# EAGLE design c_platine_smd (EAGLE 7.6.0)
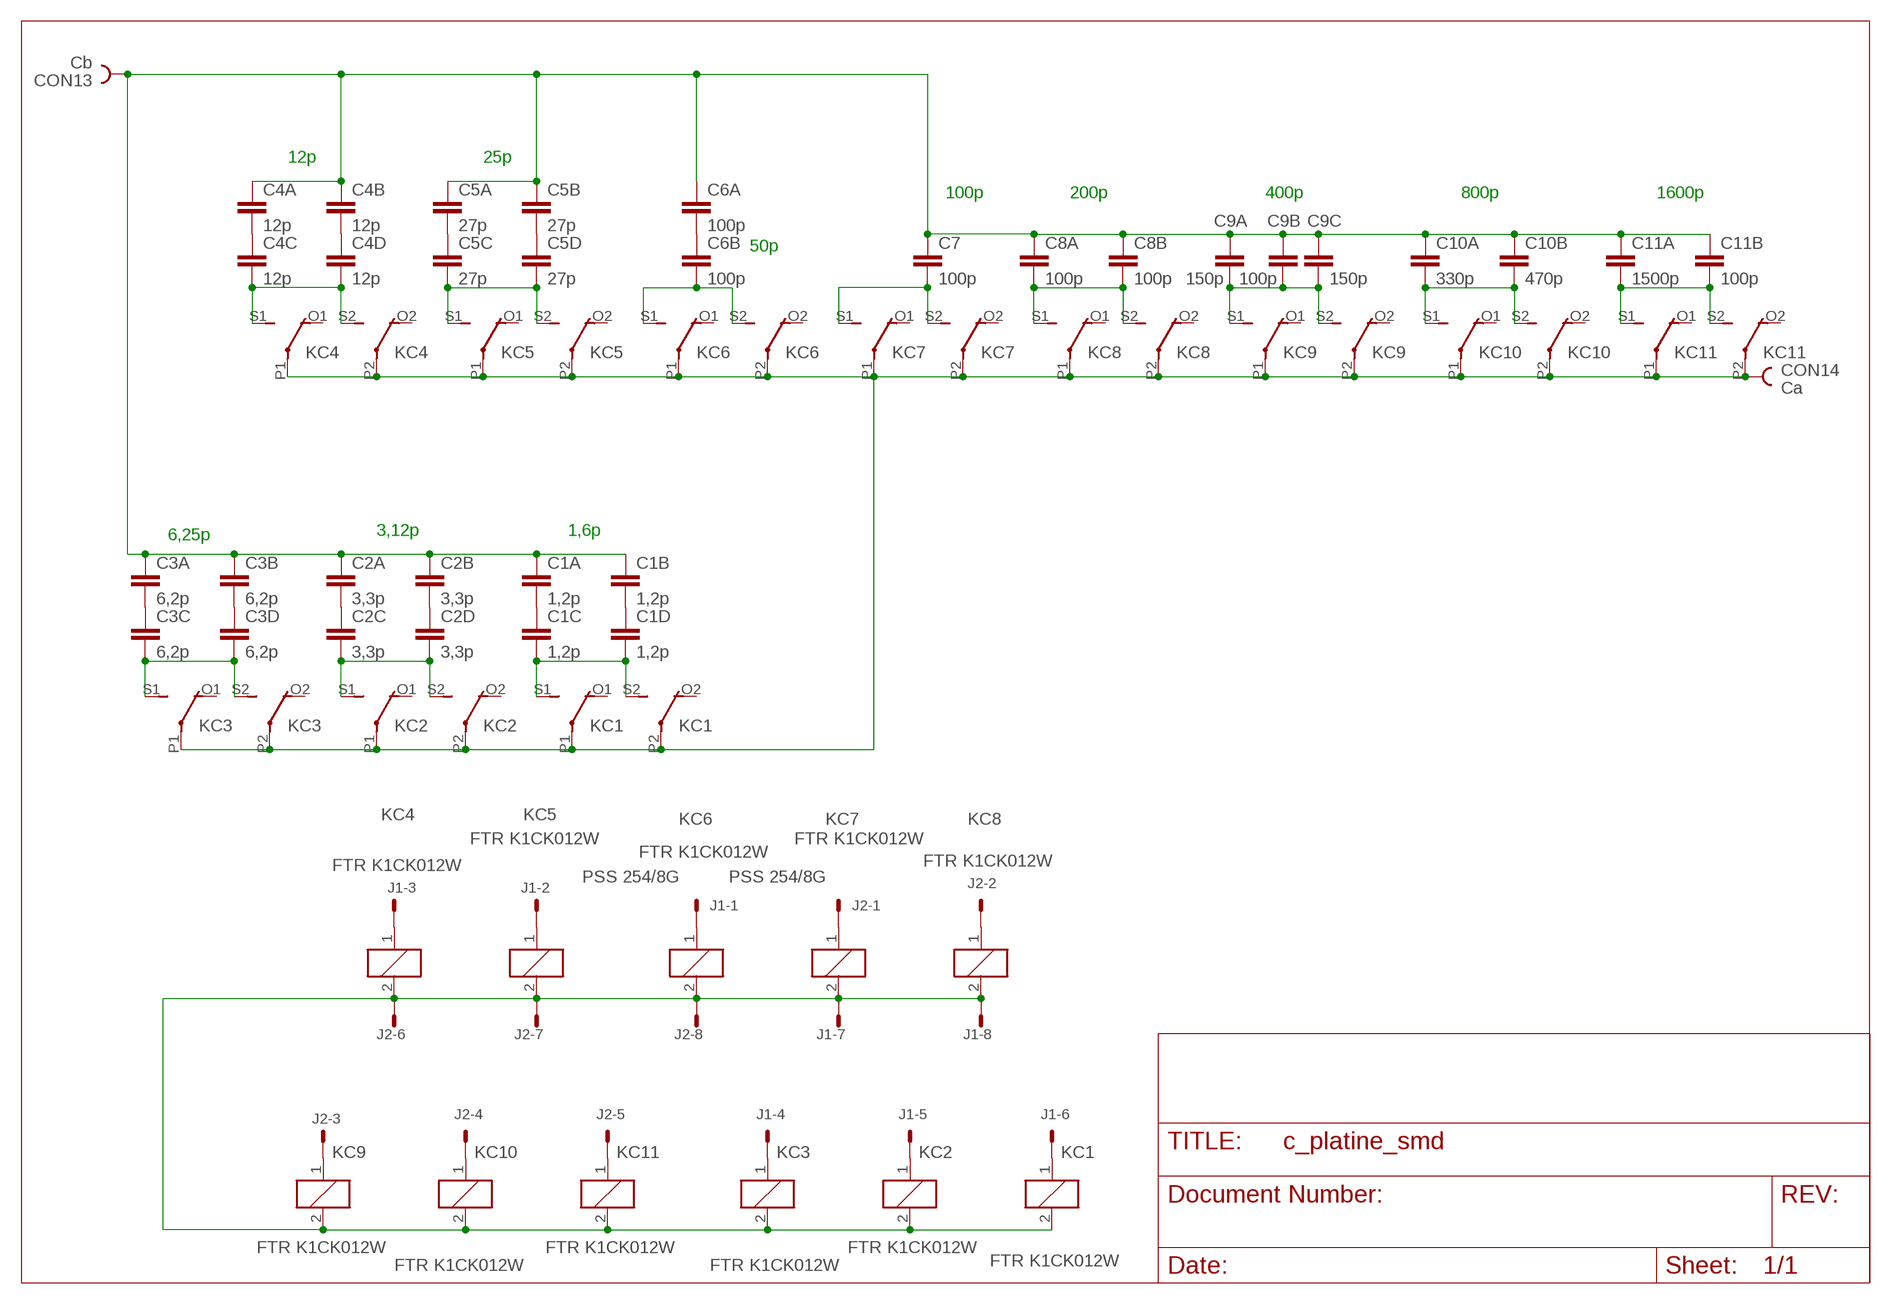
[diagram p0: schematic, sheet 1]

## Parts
C1A  1,2p  C-EUC1812K  [C1812K]
C1B  1,2p  C-EUC1812K  [C1812K]
C1C  1,2p  C-EUC1812K  [C1812K]
C1D  1,2p  C-EUC1812K  [C1812K]
C2A  3,3p  C-EUC1812K  [C1812K]
C2B  3,3p  C-EUC1812K  [C1812K]
C2C  3,3p  C-EUC1812K  [C1812K]
C2D  3,3p  C-EUC1812K  [C1812K]
C3A  6,2p  C-EUC1812K  [C1812K]
C3B  6,2p  C-EUC1812K  [C1812K]
C3C  6,2p  C-EUC1812K  [C1812K]
C3D  6,2p  C-EUC1812K  [C1812K]
C4A  12p  C-EUC1812K  [C1812K]
C4B  12p  C-EUC1812K  [C1812K]
C4C  12p  C-EUC1812K  [C1812K]
C4D  12p  C-EUC1812K  [C1812K]
C5A  27p  C-EUC1812K  [C1812K]
C5B  27p  C-EUC1812K  [C1812K]
C5C  27p  C-EUC1812K  [C1812K]
C5D  27p  C-EUC1812K  [C1812K]
C6A  100p  C-EU150-054X183  [C150-054X183]
C6B  100p  C-EU150-054X183  [C150-054X183]
C7  100p  C-EU150-054X183  [C150-054X183]
C8A  100p  C-EU150-054X183  [C150-054X183]
C8B  100p  C-EU150-054X183  [C150-054X183]
C9A  150p  C-EU150-054X183  [C150-054X183]
C9B  100p  C-EU150-054X183  [C150-054X183]
C9C  150p  C-EU150-054X183  [C150-054X183]
C10A  330p  C-EU150-054X183  [C150-054X183]
C10B  470p  C-EU150-054X183  [C150-054X183]
C11A  1500p  C-EU225-074X268  [C225-074X268]
C11B  100p  C-EU150-054X183  [C150-054X183]
CON13  Cb  PIN2_53MM  [HOLE3]
CON14  Ca  PIN2_53MM  [HOLE3]
J1  PSS 254/8G  22-27-2081-08  [6410-08]
J2  PSS 254/8G  22-27-2081-08  [6410-08]
KC1  FTR K1CK012W  4052  [F4052]
KC2  FTR K1CK012W  4052  [F4052]
KC3  FTR K1CK012W  4052  [F4052]
KC4  FTR K1CK012W  4052  [F4052]
KC5  FTR K1CK012W  4052  [F4052]
KC6  FTR K1CK012W  4052  [F4052]
KC7  FTR K1CK012W  4052  [F4052]
KC8  FTR K1CK012W  4052  [F4052]
KC9  FTR K1CK012W  4052  [F4052]
KC10  FTR K1CK012W  4052  [F4052]
KC11  FTR K1CK012W  4052  [F4052]

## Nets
N$1: CON14.1 KC1.P1(2:P) KC1.P2(3:P) KC2.P1(2:P) KC2.P2(3:P) KC3.P1(2:P) KC3.P2(3:P) KC4.P1(2:P) KC4.P2(3:P) KC5.P1(2:P) KC5.P2(3:P) KC6.P1(2:P) KC6.P2(3:P) KC7.P1(2:P) KC7.P2(3:P) KC8.P1(2:P) KC8.P2(3:P) KC9.P1(2:P) KC9.P2(3:P) KC10.P1(2:P) KC10.P2(3:P) KC11.P1(2:P) KC11.P2(3:P)
N$2: C6A.2 C6B.1
N$3: C5C.2 C5D.2 KC5.S1(2:S) KC5.S2(3:S)
N$4: C6B.2 KC6.S1(2:S) KC6.S2(3:S)
N$5: C7.2 KC7.S1(2:S) KC7.S2(3:S)
N$6: C4C.2 C4D.2 KC4.S1(2:S) KC4.S2(3:S)
N$7: C8A.2 C8B.2 KC8.S1(2:S) KC8.S2(3:S)
N$8: C9A.2 C9B.2 C9C.2 KC9.S1(2:S) KC9.S2(3:S)
N$9: C10A.2 C10B.2 KC10.S1(2:S) KC10.S2(3:S)
N$10: C11A.2 C11B.2 KC11.S1(2:S) KC11.S2(3:S)
N$11: C5A.2 C5C.1
N$12: J1.6 KC1.1
N$13: J1.5 KC2.1
N$14: J1.2 KC5.1
N$15: C4B.2 C4D.1
N$16: J1.7 J1.8 J2.6 J2.7 J2.8 KC1.2 KC2.2 KC3.2 KC4.2 KC5.2 KC6.2 KC7.2 KC8.2 KC9.2 KC10.2 KC11.2
N$17: J1.1 KC6.1
N$18: C5B.2 C5D.1
N$19: J2.1 KC7.1
N$21: J1.4 KC3.1
N$22: J2.5 KC11.1
N$23: J2.3 KC9.1
N$24: J2.4 KC10.1
N$25: J2.2 KC8.1
N$26: J1.3 KC4.1
N$27: C4A.2 C4C.1
N$28: C1A.1 C1B.1 C2A.1 C2B.1 C3A.1 C3B.1 C4A.1 C4B.1 C5A.1 C5B.1 C6A.1 C7.1 C8A.1 C8B.1 C9A.1 C9B.1 C9C.1 C10A.1 C10B.1 C11A.1 C11B.1 CON13.1
N$29: C3C.2 C3D.2 KC3.S1(2:S) KC3.S2(3:S)
N$30: C2C.2 C2D.2 KC2.S1(2:S) KC2.S2(3:S)
N$31: C1C.2 C1D.2 KC1.S1(2:S) KC1.S2(3:S)
N$32: C1B.2 C1D.1
N$33: C2B.2 C2D.1
N$34: C3B.2 C3D.1
N$35: C3A.2 C3C.1
N$36: C2A.2 C2C.1
N$37: C1A.2 C1C.1
Unconnected: KC1.O1(2:O) KC1.O2(3:O) KC2.O1(2:O) KC2.O2(3:O) KC3.O1(2:O) KC3.O2(3:O) KC4.O1(2:O) KC4.O2(3:O) KC5.O1(2:O) KC5.O2(3:O) KC6.O1(2:O) KC6.O2(3:O) KC7.O1(2:O) KC7.O2(3:O) KC8.O1(2:O) KC8.O2(3:O) KC9.O1(2:O) KC9.O2(3:O) KC10.O1(2:O) KC10.O2(3:O) KC11.O1(2:O) KC11.O2(3:O)

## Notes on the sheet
- 12p | 25p
- 100p | 200p | 400p | 800p | 1600p
- 50p
- 6,25p | 3,12p | 1,6p

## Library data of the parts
C1A C1B C1C C1D C2A C2B C2C C2D C3A C3B C3C C3D C4A C4B C4C C4D C5A C5B C5C C5D C6A C6B C7 C8A C8B C9A C9B C9C C10A C10B C11A C11B = rcl:C-EU: CAPACITOR, European symbol
CON13 CON14 = lindenau:PIN2_5
J1 J2 = con-molex:22-?-08: CONNECTOR wire to board 2.54 mm (.1 inch) pitch header; OC_FARNELL: unknown; OC_NEWARK: unknown
KC1-KC11 = relay:4052: RELAY 2 x switch, Finder; OC_FARNELL: unknown; OC_NEWARK: unknown

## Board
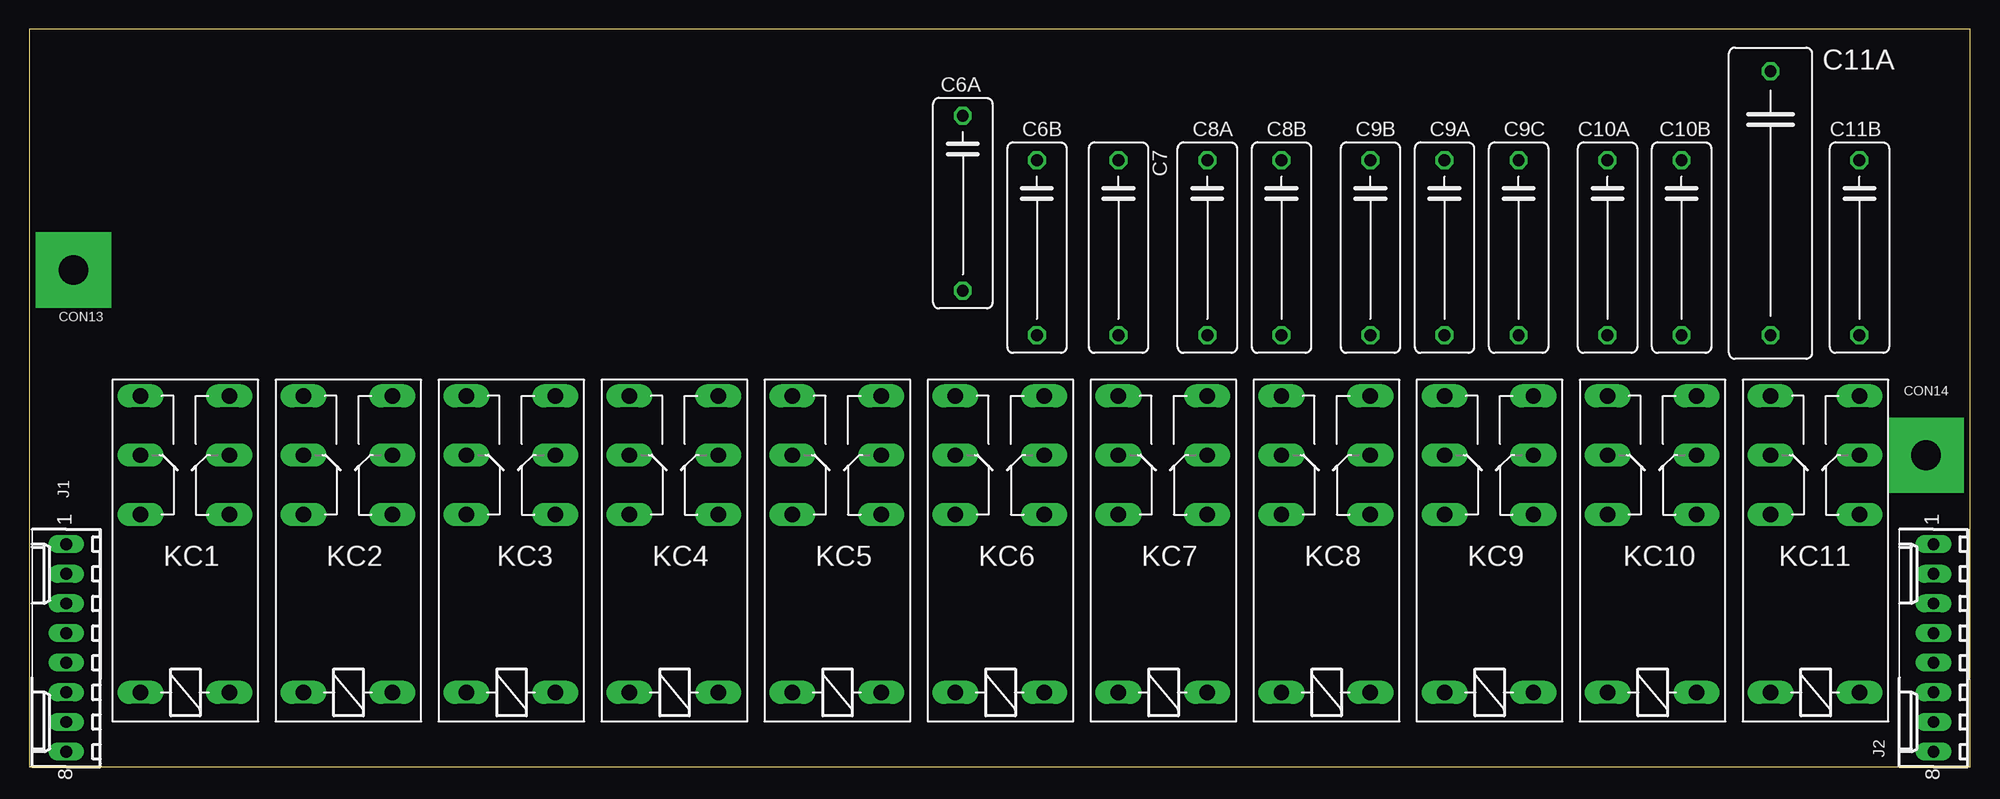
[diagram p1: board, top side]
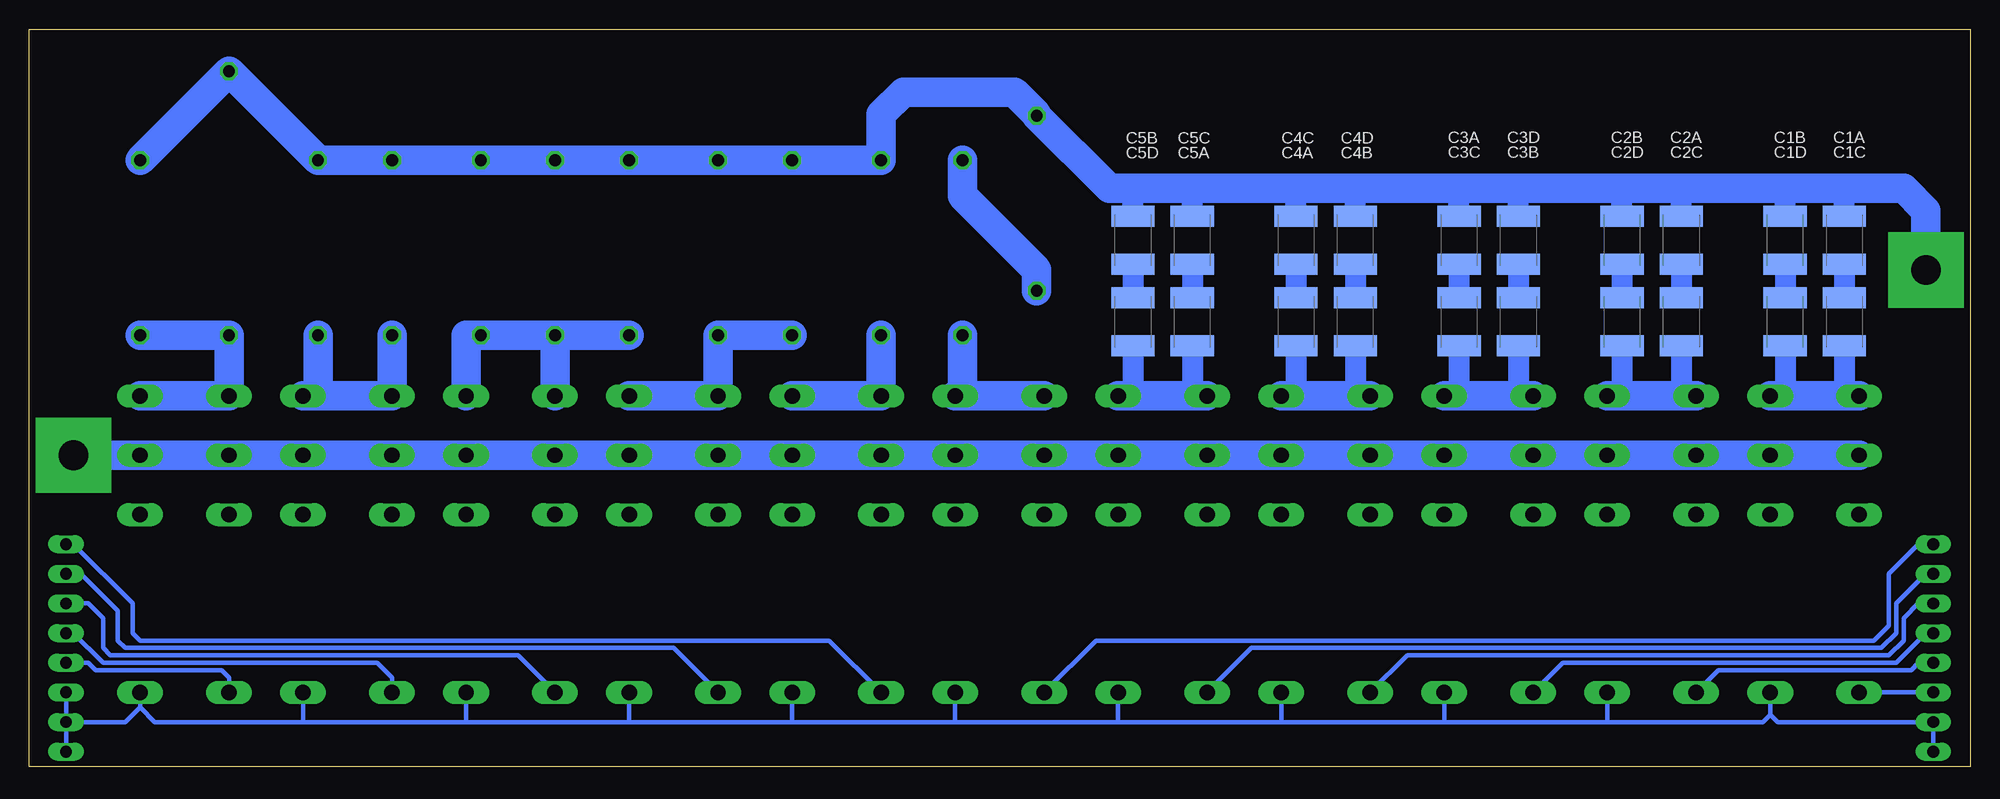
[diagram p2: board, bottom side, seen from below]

Size 166.35 x 63.17 mm. Coordinates in mm from the lower left corner, seen from the top.
Outline: 0,0 166.35,0 166.35,63.17 0,63.17 0,0
Copper layers (1*16): Top 0.035mm / dielectric 1.5mm / Bottom 0.035mm
Design rules "default": minimum track width 10mil, minimum drill 24mil, track to track 8mil, track to pad 8mil, pad to pad 8mil, via to via 8mil, smd to smd 8mil, copper to edge 40mil, drill to drill 8mil, minimum pad ring 10mil, minimum via ring 8mil, stop-mask expansion 4mil, vias tented up to drill 0mil, thermal gap 10mil

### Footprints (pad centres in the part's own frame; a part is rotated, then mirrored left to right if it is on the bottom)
C1812K = smd 1.8 x 3.7: 1 -2.05,0; 2 2.05,0
C150-054X183 = drill 1.016 octagon: 1 -7.493,0; 2 7.493,0
C225-074X268 = drill 1.016 octagon: 1 -11.303,0; 2 11.303,0
HOLE3 = drill 2.54 pad 6.452 square: 1 0,0
6410-08 = drill 1.016 long: 1 8.89,0; 2 6.35,0; 3 3.81,0; 4 1.27,0; 5 -1.27,0; 6 -3.81,0; 7 -6.35,0; 8 -8.89,0
F4052 = drill 1.321 long: 1 -3.81,3.81; 2 -3.81,-3.81; O1 11.43,-3.81; O2 11.43,3.81; P1 16.51,-3.81; P2 16.51,3.81; S1 21.59,-3.81; S2 21.59,3.81

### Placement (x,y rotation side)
C1A  10.79,45.09 270 bottom
C1B  15.88,45.09 270 bottom
C1C  10.79,38.1 270 bottom
C1D  15.88,38.1 270 bottom
C2A  24.77,45.09 270 bottom
C2B  29.85,45.09 270 bottom
C2C  24.77,38.1 270 bottom
C2D  29.85,38.1 270 bottom
C3A  43.81,45.09 270 bottom
C3B  38.73,45.09 270 bottom
C3C  43.81,38.1 270 bottom
C3D  38.73,38.1 270 bottom
C4A  57.78,45.09 270 bottom
C4B  52.7,45.09 270 bottom
C4C  57.78,38.1 270 bottom
C4D  52.7,38.1 270 bottom
C5A  66.67,45.09 270 bottom
C5B  71.75,45.09 270 bottom
C5C  66.67,38.1 270 bottom
C5D  71.75,38.1 270 bottom
C6A  80.01,48.26 270 top
C6B  86.36,44.45 270 top
C7  93.34,44.45 270 top
C8A  100.97,44.45 270 top
C8B  107.31,44.45 270 top
C9A  121.28,44.45 270 top
C9B  114.94,44.45 270 top
C9C  127.63,44.45 270 top
C10A  135.26,44.45 270 top
C10B  141.61,44.45 270 top
C11A  149.23,48.26 270 top
C11B  156.84,44.45 270 top
CON13  3.81,42.55 0 top
CON14  162.56,26.67 0 top
J1  3.17,10.16 90 top
J2  163.2,10.16 90 top
KC1  13.34,10.16 90 top
KC2  27.3,10.16 90 top
KC3  41.27,10.16 90 top
KC4  55.24,10.16 90 top
KC5  69.22,10.16 90 top
KC6  83.19,10.16 90 top
KC7  97.16,10.16 90 top
KC8  111.12,10.16 90 top
KC9  125.09,10.16 90 top
KC10  139.06,10.16 90 top
KC11  153.04,10.16 90 top

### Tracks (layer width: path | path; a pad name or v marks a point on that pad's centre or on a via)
N$1
  Bottom 2.54: KC1.P1 KC1.P2 KC2.P2 KC2.P1 KC3.P2 | KC3.P2 38.73,26.67 | KC3.P2 KC3.P1 KC4.P2 KC4.P1 KC5.P2 KC5.P1 KC6.P2 KC6.P1 KC7.P2 KC7.P1 KC8.P2 KC8.P1 KC9.P2 KC9.P1 KC10.P2 KC10.P1 KC11.P2 KC11.P1 CON14.1
N$2
  Bottom 2.54: C6A.2 80.01,42.55 86.36,48.9 C6B.1
N$3
  Bottom 1.778: C5C.2 66.67,31.75 | C5D.2 71.75,31.75
  Bottom 2.54: KC5.S2 66.67,31.75 70.48,31.75 | 70.48,31.75 71.75,31.75 KC5.S1 | 70.52,31.78 70.48,31.75
N$4
  Bottom 2.54: KC6.S2 84.45,31.75 | 84.45,31.75 86.36,31.75 | 86.36,31.75 KC6.S1 | 84.49,31.78 84.45,31.75 | C6B.2 86.36,31.75
N$5
  Bottom 2.54: C7.2 KC7.S2 KC7.S1
N$6
  Bottom 1.778: C4D.2 52.7,31.75 | C4C.2 57.78,31.75
  Bottom 2.54: KC4.S2 52.7,31.75 56.52,31.75 | 56.52,31.75 57.78,31.75 KC4.S1 | 56.55,31.78 56.52,31.75
N$7
  Bottom 2.54: C8A.2 C8B.2 KC8.S2 KC8.S1
N$8
  Bottom 2.54: C9B.2 C9A.2 | C9A.2 C9C.2 128.91,36.96 KC9.S1 | C9A.2 KC9.S2
N$9
  Bottom 2.54: 141.61,31.75 KC10.S2 C10A.2 | 141.61,31.75 KC10.S1 | 141.61,31.75 C10B.2
N$10
  Bottom 2.54: KC11.S1 KC11.S2 C11A.2 C11B.2
N$11
  Bottom 1.778: C5A.2 C5C.1
N$12
  Bottom 0.406: J1.6 KC1.1
N$13
  Bottom 0.406: J1.5 4.45,8.89 5.08,8.26 21.59,8.26 KC2.1
N$14
  Bottom 0.406: KC5.1 61.59,10.16 7.62,10.16 6.35,11.43 6.35,13.97 3.81,16.51 J1.2
N$15
  Bottom 1.778: C4B.2 C4D.1
N$16
  Bottom 0.406: KC1.2 17.14,4.45 | 17.14,4.45 17.78,3.81 31.12,3.81 | 31.12,3.81 45.08,3.81 | 45.08,3.81 59.05,3.81 | 59.05,3.81 73.02,3.81 | 73.02,3.81 86.99,3.81 | 86.99,3.81 100.97,3.81 | 100.97,3.81 114.94,3.81 | 114.94,3.81 128.91,3.81 | 128.91,3.81 142.88,3.81 | 142.88,3.81 155.58,3.81 156.84,5.08 | 156.84,5.08 KC11.2 | KC10.2 142.88,3.81 | KC9.2 128.91,3.81 | KC8.2 114.94,3.81 | KC7.2 100.97,3.81 | KC6.2 86.99,3.81 | KC5.2 73.02,3.81 | KC4.2 59.05,3.81 | KC3.2 45.08,3.81 | KC2.2 31.12,3.81 | J1.8 J1.7 16.51,3.81 17.14,4.45 | J2.8 J2.7 | J2.7 158.12,3.81 156.84,5.08 | J2.7 J2.6
N$17
  Bottom 0.406: KC6.1 74.93,10.79 8.25,10.79 6.98,12.06 6.98,16.51 4.45,19.05 J1.1
N$18
  Bottom 1.778: C5B.2 C5D.1
N$19
  Bottom 0.406: J2.1 162.56,19.05 157.48,13.97 157.48,11.43 156.84,10.79 97.79,10.79 KC7.1
N$21
  Bottom 0.406: J1.4 3.81,11.43 6.35,8.89 34.92,8.89 KC3.1
N$22
  Bottom 0.406: J2.5 161.29,8.89 160.66,8.26 149.86,8.26 149.23,7.62 KC11.1
N$23
  Bottom 0.406: J2.3 161.29,13.97 160.02,12.7 160.02,10.16 159.39,9.53 124.46,9.53 KC9.1
N$24
  Bottom 0.406: J2.4 162.56,11.43 160.02,8.89 136.53,8.89 135.26,7.62 KC10.1
N$25
  Bottom 0.406: J2.2 161.93,16.51 158.75,13.34 158.75,10.79 158.12,10.16 111.12,10.16 KC8.1
N$26
  Bottom 0.406: KC4.1 48.26,9.53 6.98,9.53 5.71,10.79 5.71,12.7 4.45,13.97 J1.3
N$27
  Bottom 1.778: C4A.2 C4C.1
N$28
  Bottom 1.778: C1A.1 10.79,49.53 | C1B.1 15.88,49.53 | C2A.1 24.77,49.53 | C2B.1 29.85,49.53 | C3B.1 38.73,49.53 | C3A.1 43.81,49.53 | C4B.1 52.7,49.53 | C4A.1 57.78,49.53 | C5A.1 66.67,49.53 | C5B.1 71.75,49.53
  Bottom 2.54: C11B.1 C11A.1 C10B.1 C10A.1 C9C.1 C9A.1 C9B.1 C8B.1 C8A.1 C7.1 93.34,55.88 91.44,57.78 81.91,57.78 80.01,55.88 C6A.1 73.79,49.53 71.75,49.53 66.67,49.53 57.78,49.53 52.7,49.53 43.81,49.53 38.73,49.53 29.85,49.53 24.77,49.53 15.88,49.53 10.79,49.53 5.71,49.53 3.81,47.62 CON13.1
N$29
  Bottom 1.778: C3D.2 38.73,31.75 | C3C.2 43.81,31.75
  Bottom 2.54: KC3.S2 38.73,31.75 43.81,31.75 KC3.S1
N$30
  Bottom 1.778: C2C.2 24.77,31.75 | C2D.2 29.85,31.75
  Bottom 2.54: KC2.S2 24.77,31.75 29.85,31.75 KC2.S1
N$31
  Bottom 1.778: C1C.2 10.79,31.75 | C1D.2 15.88,31.75
  Bottom 2.54: KC1.S2 10.79,31.75 15.88,31.75 KC1.S1
N$32
  Bottom 1.778: C1B.2 C1D.1
N$33
  Bottom 1.778: C2B.2 C2D.1
N$34
  Bottom 1.778: C3B.2 C3D.1
N$35
  Bottom 1.778: C3A.2 C3C.1
N$36
  Bottom 1.778: C2A.2 C2C.1
N$37
  Bottom 1.778: C1A.2 C1C.1

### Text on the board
tDocu: 50p | 100p | 200p | 400p | 800p | 1600p | 1,6p | 3,12p | 6,3p | 12,5p | 25p | KC6 | KC7 | KC5 | KC8 | KC4 | KC9 | KC3 | KC10 | KC2 | KC11 | KC1 | 12V | 12V | 12V | 12V | 12V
